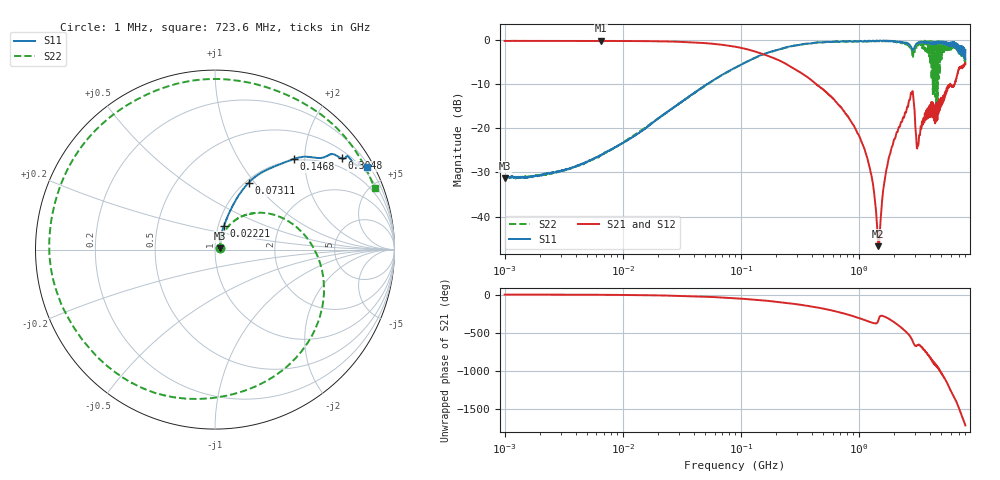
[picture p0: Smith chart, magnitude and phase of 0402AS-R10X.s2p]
!s-Parameter Generated by FASTRON Sdn. Bhd.
!FASTRON P/N : 0402AS-R10X
!Keysight Technologies: E5071C_MY46733604_B.14.02
!Date: Mon Dec 01 10:48:38 2025
!Version  :Rev00  Mon Dec 01 10:48:38 2025
!Data & Calibration Information:
!Freq  S11:SOLT2(ON)  S21:SOLT2(ON)  S12:SOLT2(ON)  S22:SOLT2(ON)
!PortZ  Port1:50+j0  Port2:50+j0
!When reading reference impedance value at option line is always used.
! Remarks : This data is being provided solely for informational purposes.
# Hz S dB R 50
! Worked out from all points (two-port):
!   1601 points, 1 MHz to 8 GHz, reference 50 ohm
!   highest |S21| = -0.20 dB at 6.532 MHz (marker M1); lowest = -46.7 dB at 1.466 GHz (marker M2)
!   |S21| within 3 dB of the highest: start of sweep to 152.8 MHz
!   lowest |S11| = -31.3 dB at 1.013 MHz (marker M3), VSWR 1.06, Z = 52.7 + j0.69 ohm
!   |S11| at or under -10 dB: start of sweep to 51.81 MHz
!   |S22| runs from -31.4 to -0.2 dB; largest |S21 - S12| = 0.0093
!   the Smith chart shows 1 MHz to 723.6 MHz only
!   S11 on the Smith chart (normalised r, x): 1 MHz: 1.05, +0.01; 22.21 MHz: 1.07, +0.29; 73.11 MHz: 1.03, +0.93; 146.8 MHz: 0.97, +1.77; 304.8 MHz: 0.70, +2.96; 723.6 MHz: 0.30, +3.89
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1000000  -31.20 13.6  -0.24 -0.6  -0.24 -0.6  -31.10 13.7
1013202  -31.30 13.9  -0.25 -0.6  -0.24 -0.6  -31.20 14.1
4479405  -28.10 45.5  -0.25 -2.7  -0.24 -2.7  -28.20 44.2
6531720  -26.20 54.2  -0.20 -3.8  -0.20 -3.8  -26.20 52.5
2.00676e7  -17.80 69.1  -0.34 -11.9  -0.34 -11.8  -17.80 61.1
2.221136e7  -16.90 69.3  -0.35 -13.2  -0.35 -13.1  -16.90 60.5
7.310609e7  -7.60 63.3  -1.19 -40.8  -1.19 -40.7  -7.64 25.1
8.994653e7  -6.29 59.8  -1.56 -49.1  -1.55 -49.1  -6.30 13.1
1.467862e8  -3.50 49.1  -3.04 -74.5  -3.03 -74.5  -3.55 -24.6
3.048452e8  -1.20 35.7  -7.04 -130.0  -7.03 -130.0  -1.18 -120.0
4.006501e8  -0.79 31.5  -9.22 -159.0  -9.20 -159.0  -0.73 -173.0
7.235966e8  -0.32 28.7  -15.60 117.0  -15.60 117.0  -0.42 21.1
9.405027e8  -0.28 32.0  -20.20 64.7  -20.20 64.6  -0.38 -88.4
1.131415e9  -0.21 36.3  -25.20 22.1  -25.20 22.0  -0.38 178.0
1.465558e9  -0.32 47.1  -46.70 21.5  -46.70 21.8  -0.23 21.2
1.7949e9  -0.21 56.6  -26.70 41.5  -26.70 41.4  -0.38 -140.0
2.222796e9  -0.48 65.0  -19.70 -58.8  -19.70 -58.8  -0.43 8.4
2.604275e9  -0.77 73.5  -15.20 -154.0  -15.10 -154.0  -0.90 178.0
3.000426e9  -1.39 95.4  -18.60 46.5  -18.60 46.3  -1.65 5.2
3.365624e9  -0.51 101.0  -19.80 34.3  -19.80 33.9  -1.43 164.0
3.710194e9  -0.74 109.0  -17.10 -30.8  -17.00 -31.2  -0.34 20.8
8e9  -2.34 -114.0  -5.45 82.1  -5.47 81.7  -4.22 115.0
